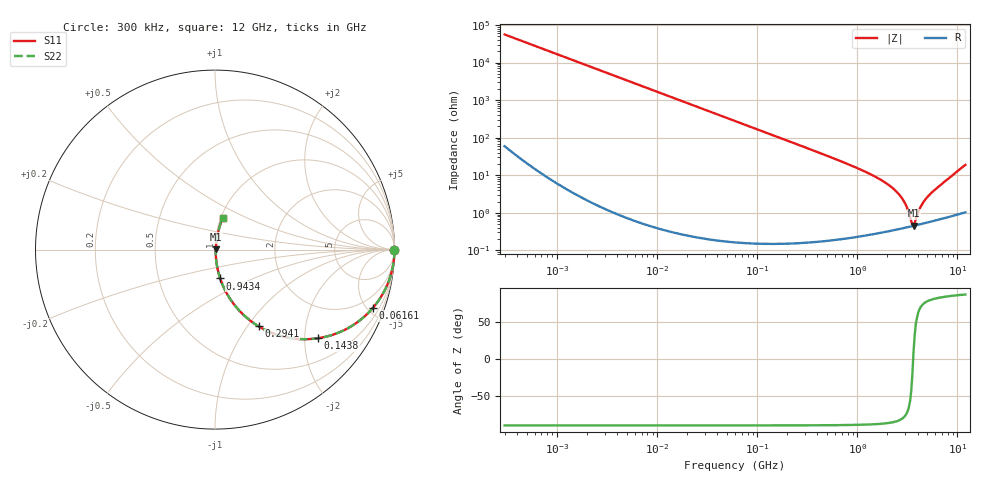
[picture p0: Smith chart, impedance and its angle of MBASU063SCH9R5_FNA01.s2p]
! MBASU063SCH9R5_FNA01  S-PARAMETER MODEL  ( General Type )
! Model Generated by TAIYO YUDEN Corporation (http://www.ty-top.com)
! Version 1.0
! TAIYO YUDEN Control No. 130801
! Copyright(c) 2013 TAIYO YUDEN CO.,LTD. All Rights Reserved.
! Product Description (link to TY-COMPAS)
! https://ds.yuden.co.jp/TYCOMPAS/or/detail?pn=MBASU063SCH9R5DFNA01&u=M
! Products Name : Multilayer Ceramic Capacitors
! Characteristics :
!  Capacitance : 9.5 pF , Rated Voltage : 50V , TCC : CH / C0H
!  Case Size : 0.6 x 0.3 / 0.024 x 0.012 [mm/inch] , Thickness : 0.3 / 0.012 [mm/inch]
!  (Conditions: Temperature = 25 degC , DC Bias Current/Voltage = 0A / 0V)
! External Node Assignments :
!  1  o---| |---o  2
! GND o---------o GND
! Frequency Range : 0.3MHz  -  12000MHz  [ 401 STEP ]
# MHz S RI R 50
! Freq[MHz].  S11 Real  S11 Imag  S21 Real  S21 Imag  S12 Real  S12 Imag  S22 Real  S22 Imag
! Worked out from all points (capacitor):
!   401 points, 300 kHz to 12 GHz, reference 50 ohm
!   read as one part in series: C = 9.5 pF near 316.3 kHz
!   lowest |Z| = 457 mohm at 3.643 GHz (marker M1)
!   series resonance near 3.612 GHz, so ESL is about 200 pH
!   S11 on the Smith chart (normalised r, x): 300 kHz: open; 61.61 MHz: 1.00, -5.44; 143.8 MHz: 1.00, -2.33; 294.1 MHz: 1.00, -1.13; 943.4 MHz: 1.00, -0.33; 12 GHz: 1.02, +0.38
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0.3  1 -0.00179  5.1e-06 0.00179  5.1e-06 0.00179  1 -0.00179
1.769972  0.9999 -0.0106  0.000114 0.0106  0.000114 0.0106  0.9999 -0.0106
10.44266  0.9961 -0.0621  0.00388 0.0621  0.00388 0.0621  0.9961 -0.0621
26.39317  0.9758 -0.1536  0.0242 0.1536  0.0242 0.1536  0.9758 -0.1536
60  0.8862 -0.3172  0.1138 0.3172  0.1138 0.3172  0.8862 -0.3172
61.61074  0.8808 -0.3238  0.1192 0.3238  0.1192 0.3238  0.8808 -0.3238
94.13233  0.7598 -0.4268  0.2402 0.4268  0.2402 0.4268  0.7598 -0.4268
143.8206  0.5751 -0.4937  0.4249 0.4937  0.4249 0.4937  0.5751 -0.4937
294.0765  0.2434 -0.4277  0.7566 0.4277  0.7566 0.4277  0.2434 -0.4277
353.9943  0.1811 -0.3834  0.8189 0.3834  0.8189 0.3834  0.1811 -0.3834
943.3804  0.0287 -0.1604  0.9713 0.1604  0.9713 0.1604  0.0287 -0.1604
1519.776  0.0109 -0.0895  0.9891 0.0895  0.9891 0.0895  0.0109 -0.0895
2088.533  0.00607 -0.0529  0.9939 0.0529  0.9939 0.0529  0.00607 -0.0529
2795.104  0.0044 -0.0238  0.9956 0.0238  0.9956 0.0238  0.0044 -0.0238
3107.553  0.00426 -0.0139  0.9957 0.0139  0.9957 0.0139  0.00426 -0.0139
3454.93  0.00436 -0.00406  0.9956 0.00406  0.9956 0.00406  0.00436 -0.00406
3642.919  0.00448 0.000765  0.9955 -0.000765  0.9955 -0.000765  0.00448 0.000765
3740.715  0.00457 0.00283  0.9954 -0.00283  0.9954 -0.00283  0.00457 0.00283
4385.161  0.00527 0.0151  0.9947 -0.0151  0.9947 -0.0151  0.00527 0.0151
5006.236  0.00614 0.0254  0.9939 -0.0254  0.9939 -0.0254  0.00614 0.0254
6879.757  0.0099 0.0554  0.9901 -0.0554  0.9901 -0.0554  0.0099 0.0554
12000  0.0435 0.1786  0.9565 -0.1786  0.9565 -0.1786  0.0435 0.1786
